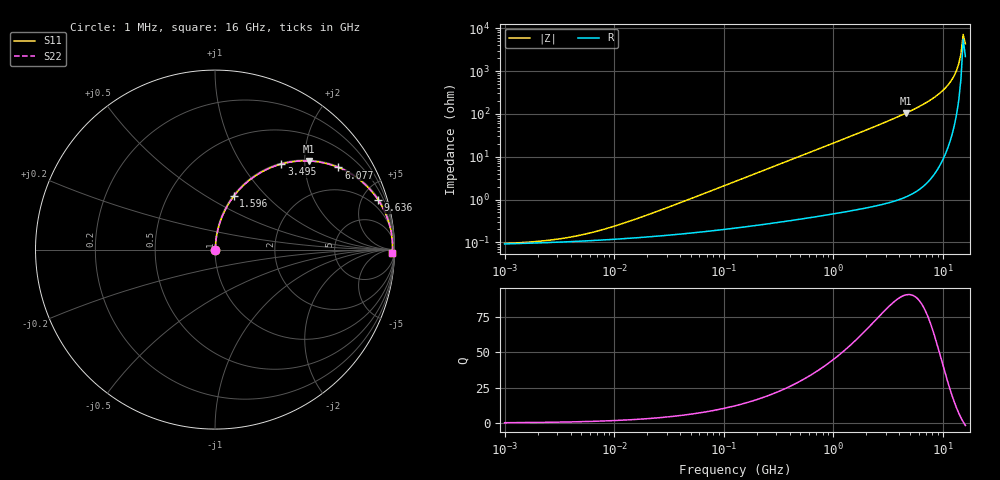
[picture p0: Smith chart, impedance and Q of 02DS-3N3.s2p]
# MHz S MA R 50
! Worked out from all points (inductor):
!   211 points, 1 MHz to 16 GHz, reference 50 ohm
!   read as one part in series: L = 3.3 nH near 20.01 MHz
!   highest Q = 90.8 at 4.609 GHz (marker M1), where L = 3.62 nH
!   self-resonance near 15.28 GHz
!   S11 on the Smith chart (normalised r, x): 1 MHz: 1.00, +0.00; 1.596 GHz: 1.01, +0.67; 3.495 GHz: 1.02, +1.53; 6.077 GHz: 1.03, +2.98; 9.636 GHz: 1.14, +6.52; 16 GHz: 45, -75
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1  0.0009422 12.7  0.9991 -0.0  0.9991 -0.0  0.0009422 12.7
2.51416  0.001118 27.7  0.999 -0.0  0.999 -0.0  0.001118 27.7
5.25662  0.001529 45.3  0.9989 -0.1  0.9989 -0.1  0.001529 45.3
10.4954  0.002477 61.2  0.9988 -0.1  0.9988 -0.1  0.002477 61.2
26.3872  0.005644 75.2  0.9986 -0.3  0.9986 -0.3  0.005644 75.2
132.458  0.02748 83.9  0.9974 -1.6  0.9974 -1.6  0.02748 83.9
664.915  0.1364 80.5  0.9868 -7.8  0.9868 -7.8  0.1364 80.5
1596.39  0.3157 70.6  0.9435 -18.4  0.9435 -18.4  0.3157 70.6
2308.32  0.4373 63.3  0.8932 -25.9  0.8932 -25.9  0.4373 63.3
3187.38  0.5648 54.9  0.8184 -34.4  0.8184 -34.4  0.5648 54.9
3495.2  0.6035 52.2  0.7903 -37.1  0.7903 -37.1  0.6035 52.2
4608.83  0.7197 43.3  0.6864 -46.0  0.6864 -46.0  0.7197 43.3
6077.26  0.8258 33.7  0.5545 -55.7  0.5545 -55.7  0.8258 33.7
7652.55  0.8979 25.3  0.4278 -63.9  0.4278 -63.9  0.8979 25.3
9636.16  0.9501 16.9  0.2916 -71.8  0.2916 -71.8  0.9501 16.9
11587.3  0.9763 10.3  0.1792 -77.3  0.1792 -77.3  0.9763 10.3
12706.4  0.9841 7.0  0.1226 -79.1  0.1226 -79.1  0.9841 7.0
13305.8  0.9867 5.4  0.09427 -79.2  0.09427 -79.2  0.9867 5.4
13933.5  0.9884 3.8  0.0661 -78.0  0.0661 -78.0  0.9884 3.8
14590.9  0.9892 2.1  0.03836 -72.7  0.03836 -72.7  0.9892 2.1
15279.2  0.9892 0.5  0.01382 -38.2  0.01382 -38.2  0.9892 0.5
16000  0.9882 -1.1  0.02286 58.4  0.02286 58.4  0.9882 -1.1
